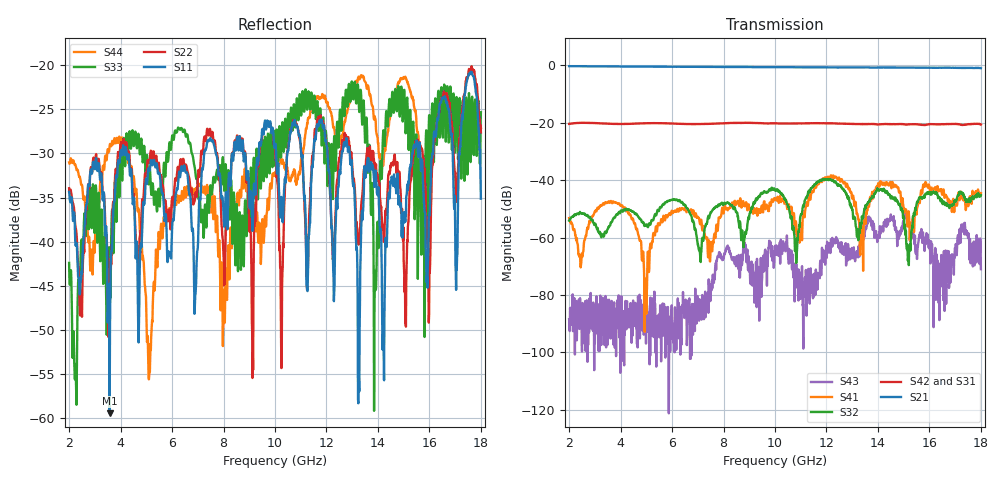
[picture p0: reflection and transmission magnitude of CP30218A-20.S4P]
! Amtery
! Email: info@amtery.com
! Phone: 886-2-2883-7839
! Model Number: CP30218A-20
! 4-port S-parameter measurement data for Dual-Directional Coupler
! Frequency Range: 2 GHz to 18 GHz
! Port 1: Input
! Port 2: Output
! Port 3: Coupled Forward
! Port 4: Coupled Reverse
# Hz S dB R 50
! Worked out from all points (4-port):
!   1281 points, 2 GHz to 18 GHz, reference 50 ohm
!   strongest paths, dB at 2 GHz, 6 GHz, 10 GHz, 14 GHz, 18 GHz:
!     S21: -0.3, -0.5, -0.6, -0.7, -1.0
!     S42: -20.4, -20.3, -20.2, -20.6, -20.6
!     S31: -20.5, -20.3, -20.2, -20.6, -20.7
!     S32: -54.1, -46.9, -43.5, -43.1, -45.3
!     S41: -53.2, -50.9, -46.9, -41.3, -44.5
!     S43: -88.4, -88.7, -62.9, -59.3, -71.0
!   lowest |S11| = -59.5 dB at 3.575 GHz (marker M1), VSWR 1.00, Z = 49.9 + j0.0227 ohm
!   |S11| at or under -10 dB: start of sweep to end of sweep
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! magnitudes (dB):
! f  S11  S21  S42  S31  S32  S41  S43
! 2 GHz  -34.4  -0.3  -20.4  -20.5  -54.1  -53.2  -88.4
! 3.575 GHz  -59.5  -0.4  -20.4  -20.5  -55.9  -47.9  -85.3
! 4.963 GHz  -33.7  -0.4  -20.2  -20.3  -55.5  -74.9  -89.8
! 6.362 GHz  -31.5  -0.5  -20.4  -20.5  -47.7  -50.2  -97.4
! 14.15 GHz  -43.5  -0.7  -20.4  -20.5  -43.4  -41.2  -56.5
! 15.19 GHz  -33.2  -0.8  -20.6  -20.7  -66.3  -50.9  -54.3
! 18 GHz  -35.1  -1.0  -20.6  -20.7  -45.3  -44.5  -71.0
